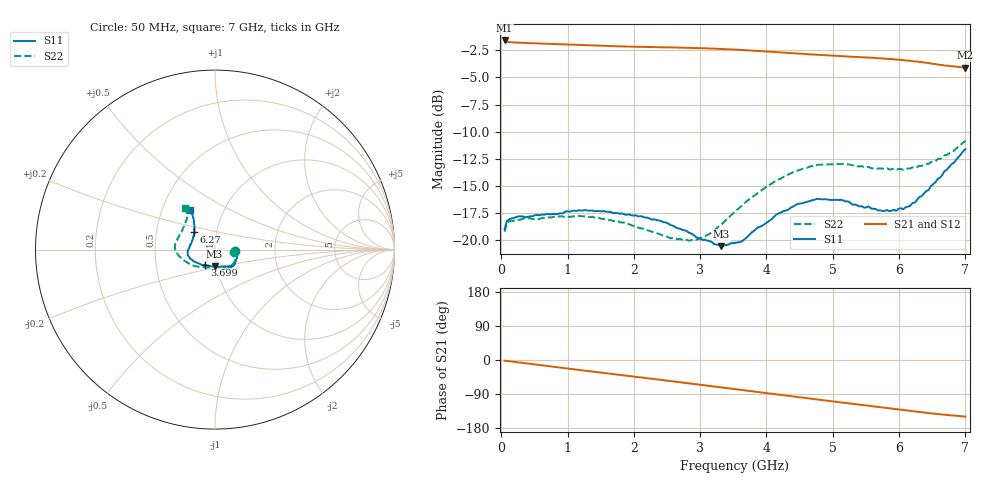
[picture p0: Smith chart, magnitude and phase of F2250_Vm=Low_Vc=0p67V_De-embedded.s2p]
! Integrated Device Technology
! Corporate Headquarters
! 6024 Silver Creek Valley Road
! San Jose, CA 95138  USA
! Phone:  1-408-284-8200
! Toll Free:  1-800-223-1366
! Webpage:  http://www.idt.com/
! Timing and RF Division
! 515 Groton Road, Suite 102
! Westford, MA 01886-6024
! Device:  F2250
! Description: Voltage Variable RF Attenuator
! Frequency:  50.0 -  6000.00 MHz
! Package:  3x3 mm Thin QFN Plastic Package: 16 pin
! Ports:  2 RF, 3 DC
!  Pin  1  = GND
!  Pin  2  = NC
!  Pin  3  = RF1  = Port 1
!  Pin  4  = NC
!  Pin  5  = GND
!  Pin  6  = GND
!  Pin  7  = GND
!  Pin  8  = GND
!  Pin  9  = NC
!  Pin 10  = RF2  = Port 2
!  Pin 11  = NC
!  Pin 12  = GND
!  Pin 13  = GND
!  Pin 14  = VCNTRL
!  Pin 15  = VDD
!  Pin 16  = VMODE
! Vcntrl:  0.670 Volts
! Vmode:  +0.000 Volts
! Vdd:  +3.30  Volts
! Current:  1.146 mA
! Data:  The device was measured on a the F2250 evaluation board which has
!  individual transmission lines to the RF pins.  Data was collected
!  using a calibrated network analyzer.  The evaluation board was
!  de-embedded using a TRL calibration technique.
!  The reference plane is the edge of the package pin.
! Misc:  SN 10
!  Action Tracker AT0258
! Date Measured:  2014-11-26
! Date:  2015-10-15  MJV
! Note:
!  Integrated Device Technology supplies this data as a sample of measured
!  data at the package pin for this product.  Your particular data for this
!  product may vary.
!  Data was taken at 25 degrees C.
!  Integrated Device Technology reserves the right to change this data at anytime.
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# GHz S dB R 50
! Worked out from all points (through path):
!   201 points, 50 MHz to 7 GHz, reference 50 ohm
!   highest |S21| = -1.58 dB at 50 MHz (marker M1); lowest = -4.1 dB at 7 GHz (marker M2)
!   group delay of S21, straight-line fit = 60 ps
!   lowest |S11| = -20.6 dB at 3.317 GHz (marker M3), VSWR 1.21, Z = 48.9 - j9.22 ohm
!   |S11| at or under -10 dB: start of sweep to end of sweep
!   |S22| runs from -20.1 to -10.9 dB; largest |S21 - S12| = 0.00071
!   S11 on the Smith chart (normalised r, x): 50 MHz: 1.25, -0.02; 3.699 GHz: 0.88, -0.15; 6.27 GHz: 0.78, +0.16; 7 GHz: 0.69, +0.33
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0.05  -19.01 -4.6  -1.58 -1.9  -1.58 -1.9  -19.24 -6.1
0.08475  -18.24 -5.0  -1.69 -2.5  -1.69 -2.5  -18.45 -6.0
0.15425  -18.01 -6.9  -1.75 -4.0  -1.75 -4.0  -18.22 -7.9
0.64075  -17.68 -22.8  -1.87 -14.7  -1.88 -14.7  -17.99 -27.6
1.2315  -17.29 -39.0  -2.02 -27.5  -2.02 -27.5  -17.83 -49.4
1.75275  -17.53 -45.8  -2.12 -38.5  -2.12 -38.5  -18.22 -60.5
2.37825  -18.21 -49.6  -2.21 -51.7  -2.20 -51.7  -19.45 -72.2
2.552  -18.63 -52.5  -2.22 -55.5  -2.22 -55.5  -19.85 -78.2
2.93425  -19.72 -65.0  -2.28 -63.9  -2.28 -63.9  -20.01 -98.1
3.14275  -20.12 -77.9  -2.32 -68.5  -2.33 -68.5  -19.44 -112.6
3.3165  -20.58 -91.6  -2.37 -72.5  -2.36 -72.5  -18.60 -123.5
3.525  -20.28 -108.7  -2.42 -77.1  -2.43 -77.1  -17.41 -135.4
3.69875  -19.79 -123.1  -2.48 -81.0  -2.49 -81.0  -16.45 -143.8
4.1505  -17.65 -148.0  -2.67 -90.9  -2.67 -91.0  -14.52 -163.2
4.7065  -16.32 -166.7  -2.88 -103.0  -2.88 -103.0  -13.19 -178.4
5.1235  -16.29 -176.9  -3.03 -111.9  -3.03 -111.9  -13.00 172.3
5.471  -17.02 172.4  -3.14 -119.3  -3.14 -119.3  -13.29 164.8
5.85325  -17.35 158.1  -3.29 -127.5  -3.29 -127.5  -13.49 155.0
6.06175  -17.17 149.0  -3.39 -132.0  -3.40 -132.0  -13.53 148.9
6.27025  -16.33 139.1  -3.53 -136.5  -3.53 -136.5  -13.27 142.2
6.61775  -14.25 126.6  -3.83 -143.2  -3.84 -143.2  -12.52 130.6
7  -11.62 121.8  -4.10 -149.4  -4.10 -149.4  -10.86 125.9
